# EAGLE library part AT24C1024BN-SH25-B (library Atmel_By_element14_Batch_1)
Two-wire Serial EEPROM
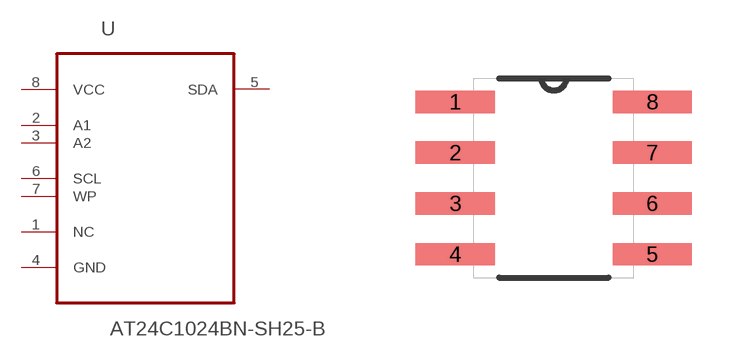
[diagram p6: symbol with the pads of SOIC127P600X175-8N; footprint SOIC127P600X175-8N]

Designator prefix U

## AT24C1024BN-SH25-B (MPN: AT24C1024BN-SH25-B; OC_FARNELL: 1455012; OC_NEWARK: 58M3811; PACKAGE: SOIC-8; SUPPLIER: Atmel)  [SOIC127P600X175-8N]
1  NC  nc
2  A1  in
3  A2  in
4  GND  pas
5  SDA
6  SCL  in
7  WP  in
8  VCC  pwr

## Footprint SOIC127P600X175-8N (pad centres in mm)
smd 1.981 x 0.559: 1 -2.464,1.905; 2 -2.464,0.635; 3 -2.464,-0.635; 4 -2.464,-1.905; 5 2.464,-1.905; 6 2.464,-0.635; 7 2.464,0.635; 8 2.464,1.905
